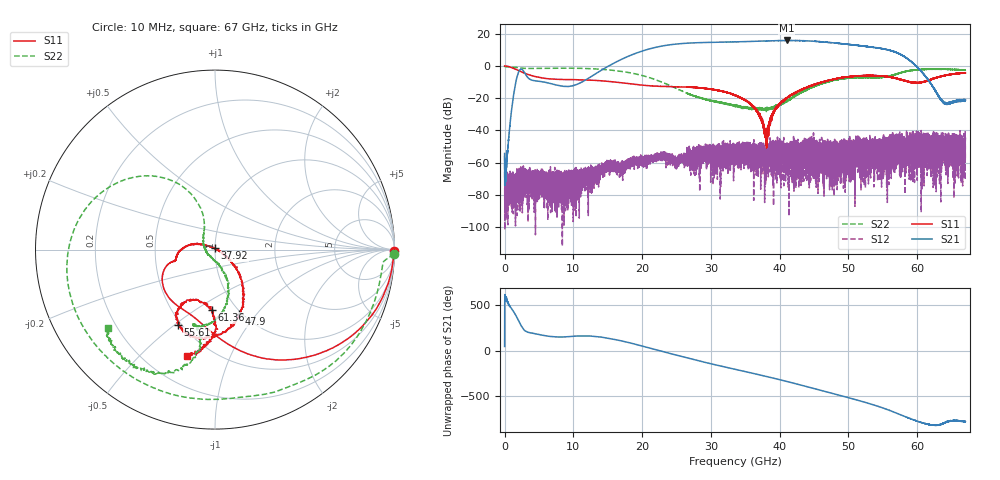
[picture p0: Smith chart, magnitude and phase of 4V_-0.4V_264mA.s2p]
! MARKI MICROWAVE INC.
! Date:  10/21/2020
! Model Number:  AMM-7210CH
! Description:  2-port Small Signal S-parameter data for AMM-7210CH
! Frequency Range:  10 MHz to 67 GHz
! Port Configuration:  PORT 1: Input
!  PORT 2: Output
! Bias Condition: Vd = +4.0V, Vg = -0.4V
! AMM-7210CH s2p files are only valid for small signal conditions (below -10 dBm input power)
# Hz S  dB  R 50
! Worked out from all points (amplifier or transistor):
!   20001 points, 10 MHz to 67 GHz, reference 50 ohm
!   highest |S21| = 15.8 dB at 41.02 GHz (marker M1)
!   |S21| within 3 dB of that: 23.54 GHz to 51.15 GHz (27.61 GHz wide, 73.9 % of centre)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
!   unconditionally stable (mu >= 1): start of sweep to end of sweep
!   at 11.17 GHz: K = 1054.43, MAG = -4.2 dB, |S12| = -68.2 dB
!   at 33.51 GHz: K = 88.22, MAG = 15.0 dB, |S12| = -60.0 dB
!   at 67 GHz: K = 327.23, MAG = -15.6 dB, |S12| = -46.3 dB
!   S11 on the Smith chart (normalised r, x): 10 MHz: open; 37.92 GHz: 1.00, +0.02; 47.9 GHz: 0.97, -0.82; 55.61 GHz: 0.48, -0.51; 61.36 GHz: 0.77, -0.58; 67 GHz: 0.38, -0.70
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1e7  -0.02 -0.4  -54.29 45.6  -55.67 -26.6  -0.02 -1.4
2.254165e9  -3.29 -63.2  -2.29 -60.8  -71.58 -40.2  -1.25 -62.5
1.117723e10  -8.59 -132.8  -10.16 163.6  -66.02 -172.7  -1.53 -168.7
1.714269e10  -10.53 -159.6  4.34 105.1  -61.32 148.2  -3.50 146.9
1.999982e10  -11.89 -164.0  9.17 51.7  -55.88 125.1  -5.96 126.7
2.234112e10  -12.68 -164.0  11.83 4.0  -54.45 108.2  -9.19 113.9
2.460538e10  -12.94 -165.9  13.36 -42.8  -58.11 83.1  -13.18 108.9
2.753954e10  -13.30 -170.6  14.28 -100.5  -66.98 110.9  -18.64 121.1
3.068472e10  -14.91 178.3  14.66 -157.8  -54.40 69.1  -21.97 147.7
3.3505e10  -18.23 166.5  14.91 153.1  -60.00 27.5  -24.30 170.2
3.792299e10  -41.47 98.7  15.43 75.8  -51.94 6.6  -27.06 -126.7
4.102463e10  -20.00 -36.2  15.77 18.5  -59.34 -76.1  -21.67 -79.3
4.274962e10  -15.47 -42.1  15.68 -15.3  -54.16 -59.2  -17.25 -69.7
4.467223e10  -12.25 -51.8  15.39 -53.8  -56.06 47.2  -13.33 -69.9
4.79045e10  -8.29 -69.3  14.21 -118.7  -48.46 -134.3  -8.91 -84.7
5.12808e10  -6.25 -91.8  12.72 171.5  -61.24 121.7  -7.21 -101.6
5.36355e10  -5.96 -105.5  11.49 119.0  -52.75 -146.7  -7.26 -106.1
5.5605e10  -6.58 -116.4  10.11 67.9  -46.17 137.2  -6.54 -100.5
5.583612e10  -6.85 -117.0  9.84 61.8  -69.94 110.7  -6.41 -100.5
5.86162e10  -9.73 -117.8  4.31 -22.4  -53.64 -32.8  -3.25 -106.6
6.136279e10  -9.45 -93.3  -7.44 -92.0  -52.52 -162.3  -2.07 -122.6
6.7e10  -4.45 -104.8  -21.12 -66.7  -46.29 103.8  -2.48 -144.0
